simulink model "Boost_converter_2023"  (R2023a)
settings: Solver=VariableStepAuto  StartTime=0.0  StopTime=0.1  MaxStep=1e-5  RelTol=1e-3
libraries: spsSeriesRLCBranchLib x3, spsVoltageMeasurementLib x2, spsCurrentMeasurementLib x1, spsDCVoltageSourceLib x1, spsDiodeLib x1, spsMosfetLib x1, simulink x1, spspowerguiLib x1

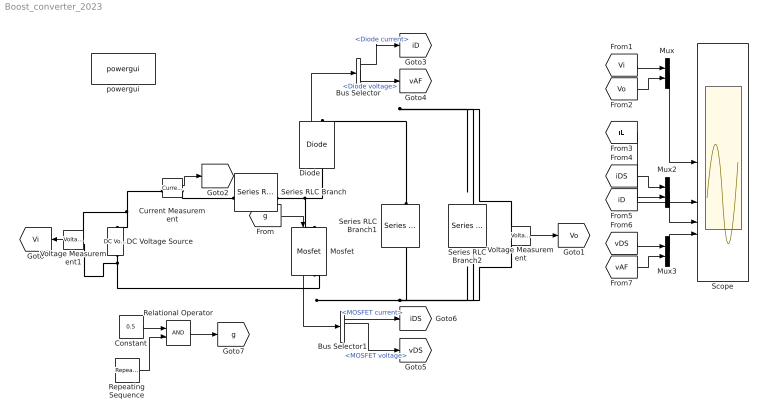
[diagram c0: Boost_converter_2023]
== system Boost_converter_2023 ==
  Bus Selector : BusSelector  OutputSignals=Diode current,Diode voltage
  Bus Selector1 : BusSelector  OutputSignals=MOSFET current,MOSFET voltage
  Constant : Constant  Value=0.5
  Current Measurement : spsCurrentMeasurementLib/Current Measurement  PhasorSimulation=off  OutputType=Complex  PSBequivalent=0
  DC Voltage Source : spsDCVoltageSourceLib/DC Voltage Source  Amplitude=100  Measurements=None
  Diode : spsDiodeLib/Diode  Ron=0.001  Lon=0  Vf=0.8  IC=0  UseSnubber=0  Rs=500  Cs=250e-9  Measurements=on
  Mosfet : spsMosfetLib/Mosfet  Ron=0.1  Lon=0  Rd=0.01  Vfd=0  IC=0  Rs=1e5  Cs=inf  Measurements=on
  Mux : Mux  Inputs=2
  Mux2 : Mux  Inputs=2
  Mux3 : Mux  Inputs=2
  Relational Operator : RelationalOperator  OutDataTypeStr=boolean  RndMeth=Simplest
  Repeating Sequence : simulink/Sources/Repeating Sequence  rep_seq_t=[0 0.000025 0.00005]  rep_seq_y=[0 1 0]
  Scope : Scope  NumInputPorts=4
  Series RLC Branch : spsSeriesRLCBranchLib/Series RLC Branch  LConnTagsString=__new0  RConnTagsString=__new0  BranchType=L  Resistance=1  Inductance=1e-3  SetiL0=off  InitialCurrent=0  Capacitance=1e-6  Setx0=off  InitialVoltage=0  Measurements=None
  Series RLC Branch1 : spsSeriesRLCBranchLib/Series RLC Branch  LConnTagsString=__new0  RConnTagsString=__new0  BranchType=C  Resistance=1  Inductance=1e-3  SetiL0=off  InitialCurrent=0  Capacitance=1e-3  Setx0=on  InitialVoltage=200  Measurements=None
  Series RLC Branch2 : spsSeriesRLCBranchLib/Series RLC Branch  LConnTagsString=__new0  RConnTagsString=__new0  BranchType=R  Resistance=20  Inductance=1e-3  SetiL0=off  InitialCurrent=0  Capacitance=1e-3  Setx0=on  InitialVoltage=200  Measurements=None
  Voltage Measurement : spsVoltageMeasurementLib/Voltage Measurement  PhasorSimulation=off  OutputType=Complex  PSBequivalent=0
  Voltage Measurement1 : spsVoltageMeasurementLib/Voltage Measurement  PhasorSimulation=off  OutputType=Complex  PSBequivalent=0
  powergui : spspowerguiLib/powergui  Priority=1  SimulationMode=Continuous  SampleTime=50e-6  frequency=60  Iterations=50  frequencyindice=0  Pbase=100e6  ErrMax=1e-4  UnitsV=kV  UnitsW=MW  buscounter=0  FunctionMessages=off  echomessages=off  EnableUseOfTLC=off  CurrentSourceSwitches=off  DisableSnubberDevices=off  DisableRonSwitches=off  DisableVfSwitches=off  DisplayEquations=off  AutomaticDiscreteSolvers=off  SolverType=Tustin/Backward Euler (TBE)  Interpol=off  ExternalGateDelay=off  methode=off  Ts=100  x0status=blocks  SPID=on  SwTol=0  HookPort=off  NonlinearTolerance=1e-4  nMaxIteration=100  ContinueOnMaxIteration=off  RestoreLinks=warning  ResistiveCurrentMeasurement=off  Frange=[0:2:500]  Ylog=off  Xlog=on  ShowGrid=off  save=off  variable=ZData  structure=0  ZoomFFT=off  StartTime=0.0  cycles=1  DisplayStyle=1  fundamental=60  FreqAxis=off  MaxFrequency=1000  frequencyindicesteady=1  RmsSteady=1  display=off
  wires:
  [g] -> Mosfet/1
  Voltage Measurement1/1 -> [Vi]
  Voltage Measurement/1 -> [Vo]
  Current Measurement/1 -> [iL]
  Diode/1 -> Bus Selector/1
  Mosfet/1 -> Bus Selector1/1
  Bus Selector/1 -> [iD]  "<Diode current>"
  Bus Selector/2 -> [vAF]  "<Diode voltage>"
  Bus Selector1/1 -> [iDS]  "<MOSFET current>"
  Bus Selector1/2 -> [vDS]  "<MOSFET voltage>"
  Mux/1 -> Scope/1
  [iL] -> Scope/2
  Mux3/1 -> Scope/4
  Mux2/1 -> Scope/3
  [Vi] -> Mux/1
  [Vo] -> Mux/2
  [iDS] -> Mux2/1
  [iD] -> Mux2/2
  [vDS] -> Mux3/1
  [vAF] -> Mux3/2
  Relational Operator/1 -> [g]
  Repeating Sequence/1 -> Relational Operator/2
  Constant/1 -> Relational Operator/1
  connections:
  Series RLC Branch/RConn1 -- Mosfet/LConn1 -- Diode/LConn1
  DC Voltage Source/LConn1 -- Voltage Measurement1/LConn2 -- Voltage Measurement/LConn2 -- Series RLC Branch2/RConn1 -- Series RLC Branch1/RConn1 -- Mosfet/RConn1
  Series RLC Branch1/LConn1 -- Voltage Measurement/LConn1 -- Series RLC Branch2/LConn1 -- Diode/RConn1
  Current Measurement/RConn1 -- Series RLC Branch/LConn1
  Current Measurement/LConn1 -- Voltage Measurement1/LConn1 -- DC Voltage Source/RConn1
